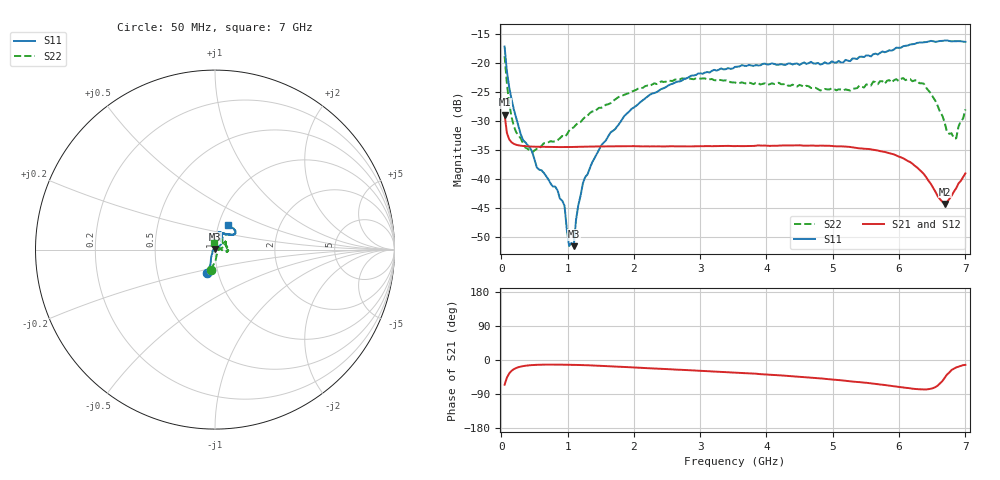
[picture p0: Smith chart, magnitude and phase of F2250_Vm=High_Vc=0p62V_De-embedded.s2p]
! Integrated Device Technology
! Corporate Headquarters
! 6024 Silver Creek Valley Road
! San Jose, CA 95138  USA
! Phone:  1-408-284-8200
! Toll Free:  1-800-223-1366
! Webpage:  http://www.idt.com/
! Timing and RF Division
! 515 Groton Road, Suite 102
! Westford, MA 01886-6024
! Device:  F2250
! Description: Voltage Variable RF Attenuator
! Frequency:  50.0 -  6000.00 MHz
! Package:  3x3 mm Thin QFN Plastic Package: 16 pin
! Ports:  2 RF, 3 DC
!  Pin  1  = GND
!  Pin  2  = NC
!  Pin  3  = RF1  = Port 1
!  Pin  4  = NC
!  Pin  5  = GND
!  Pin  6  = GND
!  Pin  7  = GND
!  Pin  8  = GND
!  Pin  9  = NC
!  Pin 10  = RF2  = Port 2
!  Pin 11  = NC
!  Pin 12  = GND
!  Pin 13  = GND
!  Pin 14  = VCNTRL
!  Pin 15  = VDD
!  Pin 16  = VMODE
! Vcntrl:  0.620 Volts
! Vmode:  +3.300 Volts
! Vdd:  +3.30  Volts
! Current:  1.279 mA
! Data:  The device was measured on a the F2250 evaluation board which has
!  individual transmission lines to the RF pins.  Data was collected
!  using a calibrated network analyzer.  The evaluation board was
!  de-embedded using a TRL calibration technique.
!  The reference plane is the edge of the package pin.
! Misc:  SN 10
!  Action Tracker AT0258
! Date Measured:  2014-11-26
! Date:  2015-10-15  MJV
! Note:
!  Integrated Device Technology supplies this data as a sample of measured
!  data at the package pin for this product.  Your particular data for this
!  product may vary.
!  Data was taken at 25 degrees C.
!  Integrated Device Technology reserves the right to change this data at anytime.
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# GHz S dB R 50
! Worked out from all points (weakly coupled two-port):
!   201 points, 50 MHz to 7 GHz, reference 50 ohm
!   highest |S21| = -28.95 dB at 50 MHz (marker M1); lowest = -44.4 dB at 6.687 GHz (marker M2)
!   lowest |S11| = -51.6 dB at 1.093 GHz (marker M3), VSWR 1.01, Z = 50 + j0.261 ohm
!   |S11| at or under -10 dB: start of sweep to end of sweep
!   |S22| runs from -35.4 to -18.8 dB; largest |S21 - S12| = 6.2e-05
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0.05  -17.17 -108.3  -28.95 -65.1  -28.95 -65.1  -18.80 -102.3
0.08475  -21.46 -107.2  -32.09 -46.3  -32.09 -46.3  -23.56 -88.3
0.15425  -26.23 -116.3  -33.69 -28.6  -33.69 -28.6  -29.33 -76.3
0.29325  -32.31 -126.8  -34.28 -17.3  -34.28 -17.3  -33.01 -47.2
0.36275  -33.69 -139.0  -34.37 -15.1  -34.37 -15.2  -34.63 -30.0
0.5365  -38.04 -154.0  -34.46 -12.7  -34.46 -12.7  -34.84 -11.0
0.84925  -42.03 170.2  -34.52 -12.2  -34.52 -12.2  -33.32 2.7
0.9535  -44.63 171.4  -34.52 -12.3  -34.52 -12.4  -32.78 6.2
1.023  -51.60 138.1  -34.51 -12.5  -34.51 -12.6  -31.70 8.0
1.0925  -51.63 83.6  -34.50 -12.8  -34.50 -12.8  -31.12 9.8
1.12725  -47.10 58.2  -34.49 -13.0  -34.49 -13.0  -30.66 8.8
1.2315  -40.74 39.1  -34.46 -13.5  -34.46 -13.5  -29.70 7.9
1.6485  -31.99 40.6  -34.40 -16.5  -34.40 -16.6  -26.93 16.9
2.37825  -24.75 46.4  -34.39 -22.9  -34.39 -23.0  -23.47 27.0
3.525  -20.67 71.6  -34.36 -33.4  -34.36 -33.4  -23.37 54.9
4.7065  -20.08 71.9  -34.25 -47.1  -34.25 -47.2  -24.32 58.7
5.2625  -19.68 53.1  -34.50 -56.2  -34.50 -56.3  -24.76 35.3
5.85325  -17.80 40.5  -35.59 -67.6  -35.59 -67.7  -22.95 6.6
6.3745  -16.41 40.9  -39.19 -77.8  -39.20 -77.8  -23.58 -10.1
6.68725  -16.12 47.8  -44.36 -47.1  -44.35 -46.9  -30.30 9.7
6.861  -16.23 54.4  -41.62 -19.7  -41.59 -19.7  -33.01 61.4
7  -16.34 62.3  -39.06 -12.8  -39.02 -13.0  -28.02 99.6
